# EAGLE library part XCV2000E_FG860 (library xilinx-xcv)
xcv2000e_fg860 edit this description Auto generated by make-symbol-device-package-bsdl.ulp Rev. 26 Source: xcv2000e_fg860.bsd
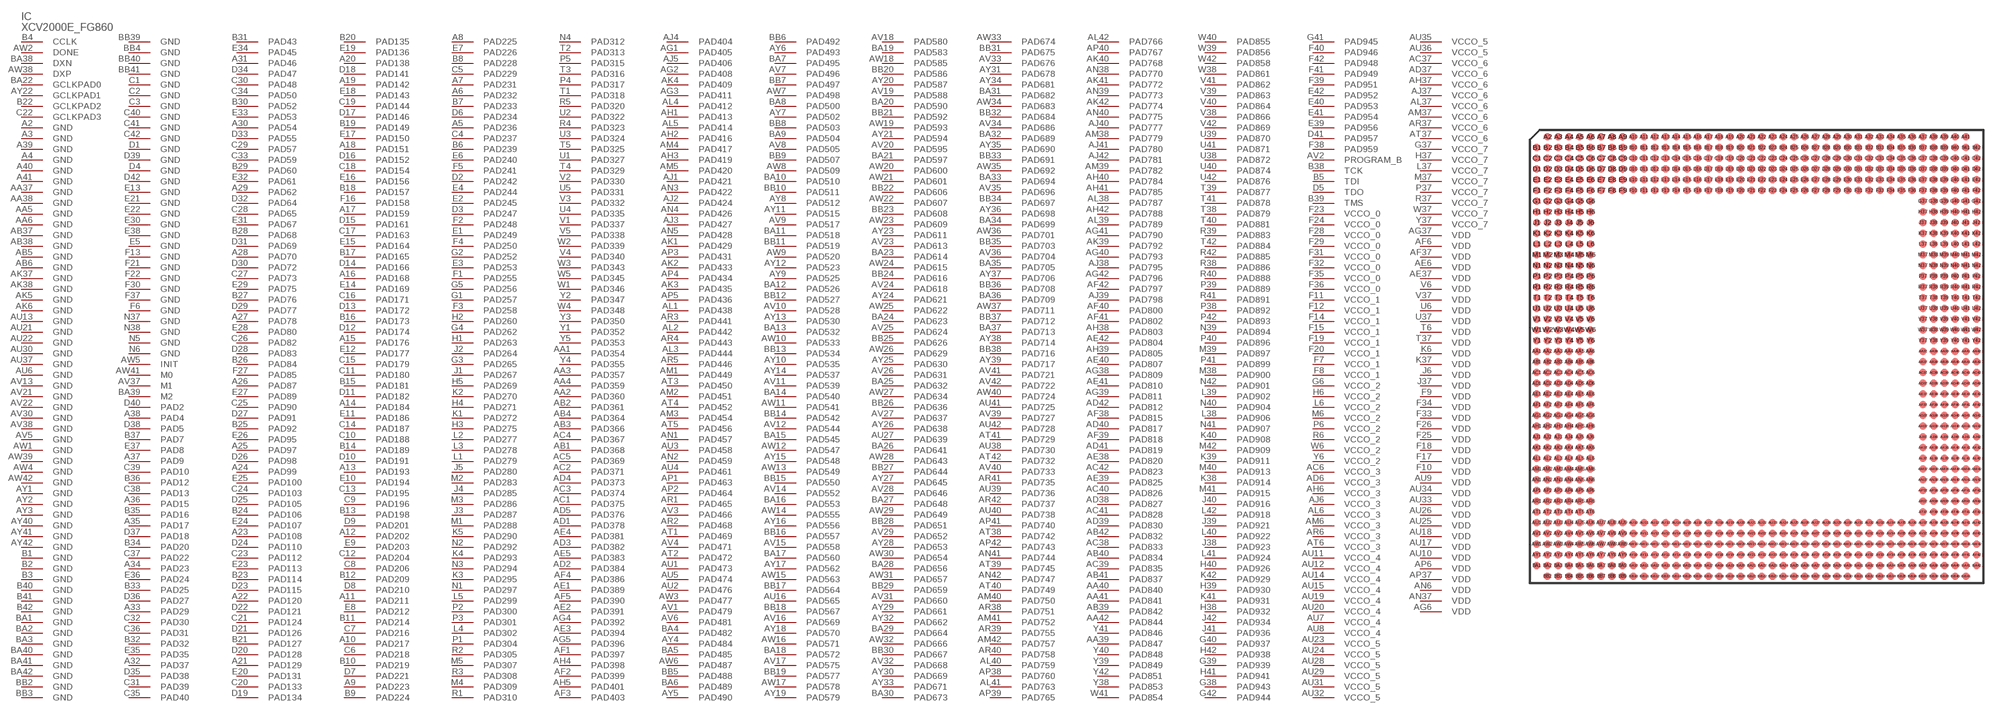
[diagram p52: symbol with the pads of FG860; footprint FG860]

Designator prefix IC

## XCV2000E_FG860 (OC_FARNELL: unknown; OC_NEWARK: unknown)  [FG860]
A2  GND  pwr
A3  GND  pwr
A4  GND  pwr
A5  PAD236
A6  PAD232
A7  PAD231
A8  PAD225
A9  PAD223
A10  PAD217
A11  PAD211
A12  PAD202
A13  PAD193
A14  PAD184
A15  PAD176
A16  PAD168
A17  PAD159
A18  PAD151
A19  PAD142
A20  PAD138
A21  PAD129
A22  PAD120
A23  PAD108
A24  PAD99
A25  PAD97
A26  PAD87
A27  PAD78
A28  PAD70
A29  PAD62
A30  PAD54
A31  PAD46
A32  PAD37
A33  PAD29
A34  PAD23
A35  PAD17
A36  PAD15
A37  PAD9
A38  PAD4
A39  GND  pwr
A40  GND  pwr
A41  GND  pwr
AA1  PAD354
AA2  PAD360
AA3  PAD357
AA4  PAD359
AA5  GND  pwr
AA6  GND  pwr
AA37  GND  pwr
AA38  GND  pwr
AA39  PAD847
AA40  PAD840
AA41  PAD841
AA42  PAD844
AB1  PAD368
AB2  PAD361
AB3  PAD366
AB4  PAD364
AB5  GND  pwr
AB6  GND  pwr
AB37  GND  pwr
AB38  GND  pwr
AB39  PAD842
AB40  PAD834
AB41  PAD837
AB42  PAD832
AC1  PAD375
AC2  PAD371
AC3  PAD374
AC4  PAD367
AC5  PAD369
AC6  VCCO_3  pwr
AC37  VCCO_6  pwr
AC38  PAD833
AC39  PAD835
AC40  PAD826
AC41  PAD828
AC42  PAD823
AD1  PAD378
AD2  PAD384
AD3  PAD382
AD4  PAD373
AD5  PAD376
AD6  VCCO_3  pwr
AD37  VCCO_6  pwr
AD38  PAD827
AD39  PAD830
AD40  PAD817
AD41  PAD819
AD42  PAD812
AE1  PAD389
AE2  PAD391
AE3  PAD394
AE4  PAD381
AE5  PAD383
AE6  VDD  pwr
AE37  VDD  pwr
AE38  PAD820
AE39  PAD825
AE40  PAD807
AE41  PAD810
AE42  PAD804
AF1  PAD397
AF2  PAD399
AF3  PAD403
AF4  PAD386
AF5  PAD390
AF6  VDD  pwr
AF37  VDD  pwr
AF38  PAD815
AF39  PAD818
AF40  PAD800
AF41  PAD802
AF42  PAD797
AG1  PAD405
AG2  PAD408
AG3  PAD411
AG4  PAD392
AG5  PAD396
AG6  VDD  pwr
AG37  VDD  pwr
AG38  PAD809
AG39  PAD811
AG40  PAD793
AG41  PAD790
AG42  PAD796
AH1  PAD413
AH2  PAD416
AH3  PAD419
AH4  PAD398
AH5  PAD401
AH6  VCCO_3  pwr
AH37  VCCO_6  pwr
AH38  PAD803
AH39  PAD805
AH40  PAD784
AH41  PAD785
AH42  PAD788
AJ1  PAD421
AJ2  PAD424
AJ3  PAD427
AJ4  PAD404
AJ5  PAD406
AJ6  VCCO_3  pwr
AJ37  VCCO_6  pwr
AJ38  PAD795
AJ39  PAD798
AJ40  PAD777
AJ41  PAD780
AJ42  PAD781
AK1  PAD429
AK2  PAD433
AK3  PAD435
AK4  PAD409
AK5  GND  pwr
AK6  GND  pwr
AK37  GND  pwr
AK38  GND  pwr
AK39  PAD792
AK40  PAD768
AK41  PAD772
AK42  PAD774
AL1  PAD438
AL2  PAD442
AL3  PAD444
AL4  PAD412
AL5  PAD414
AL6  VCCO_3  pwr
AL37  VCCO_6  pwr
AL38  PAD787
AL39  PAD789
AL40  PAD759
AL41  PAD763
AL42  PAD766
AM1  PAD449
AM2  PAD451
AM3  PAD454
AM4  PAD417
AM5  PAD420
AM6  VCCO_3  pwr
AM37  VCCO_6  pwr
AM38  PAD779
AM39  PAD782
AM40  PAD750
AM41  PAD752
AM42  PAD757
AN1  PAD457
AN2  PAD459
AN3  PAD422
AN4  PAD426
AN5  PAD428
AN6  VDD  pwr
AN37  VDD  pwr
AN38  PAD770
AN39  PAD773
AN40  PAD775
AN41  PAD744
AN42  PAD747
AP1  PAD463
AP2  PAD464
AP3  PAD431
AP4  PAD434
AP5  PAD436
AP6  VDD  pwr
AP37  VDD  pwr
AP38  PAD760
AP39  PAD765
AP40  PAD767
AP41  PAD740
AP42  PAD743
AR1  PAD465
AR2  PAD468
AR3  PAD441
AR4  PAD443
AR5  PAD446
AR6  VCCO_3  pwr
AR37  VCCO_6  pwr
AR38  PAD751
AR39  PAD755
AR40  PAD758
AR41  PAD735
AR42  PAD737
AT1  PAD469
AT2  PAD472
AT3  PAD450
AT4  PAD452
AT5  PAD456
AT6  VCCO_3  pwr
AT37  VCCO_6  pwr
AT38  PAD742
AT39  PAD745
AT40  PAD749
AT41  PAD729
AT42  PAD732
AU1  PAD473
AU2  PAD476
AU3  PAD458
AU4  PAD461
AU5  PAD474
AU6  GND  pwr
AU7  VCCO_4  pwr
AU8  VCCO_4  pwr
AU9  VDD  pwr
AU10  VDD  pwr
AU11  VCCO_4  pwr
AU12  VCCO_4  pwr
AU13  GND  pwr
AU14  VCCO_4  pwr
AU15  VCCO_4  pwr
AU16  PAD565
AU17  VDD  pwr
AU18  VDD  pwr
AU19  VCCO_4  pwr
AU20  VCCO_4  pwr
AU21  GND  pwr
AU22  GND  pwr
AU23  VCCO_5  pwr
AU24  VCCO_5  pwr
AU25  VDD  pwr
AU26  VDD  pwr
AU27  PAD639
AU28  VCCO_5  pwr
AU29  VCCO_5  pwr
AU30  GND  pwr
AU31  VCCO_5  pwr
AU32  VCCO_5  pwr
AU33  VDD  pwr
AU34  VDD  pwr
AU35  VCCO_5  pwr
AU36  VCCO_5  pwr
AU37  GND  pwr
AU38  PAD730
AU39  PAD736
AU40  PAD738
AU41  PAD725
AU42  PAD728
AV1  PAD479
AV2  PROGRAM_B  in
AV3  PAD466
AV4  PAD471
AV5  GND  pwr
AV6  PAD481
AV7  PAD496
AV8  PAD505
AV9  PAD517
AV10  PAD528
AV11  PAD539
AV12  PAD544
AV13  GND  pwr
AV14  PAD552
AV15  PAD558
AV16  PAD569
AV17  PAD575
AV18  PAD580
AV19  PAD588
AV20  PAD595
AV21  GND  pwr
AV22  GND  pwr
AV23  PAD613
AV24  PAD618
AV25  PAD624
AV26  PAD631
AV27  PAD637
AV28  PAD646
AV29  PAD652
AV30  GND  pwr
AV31  PAD660
AV32  PAD668
AV33  PAD676
AV34  PAD686
AV35  PAD696
AV36  PAD704
AV37  M1  in
AV38  GND  pwr
AV39  PAD727
AV40  PAD733
AV41  PAD721
AV42  PAD722
AW1  GND  pwr
AW2  DONE
AW3  PAD477
AW4  GND  pwr
AW5  INIT
AW6  PAD487
AW7  PAD498
AW8  PAD509
AW9  PAD520
AW10  PAD533
AW11  PAD541
AW12  PAD547
AW13  PAD549
AW14  PAD555
AW15  PAD563
AW16  PAD571
AW17  PAD578
AW18  PAD585
AW19  PAD593
AW20  PAD600
AW21  PAD601
AW22  PAD607
AW23  PAD609
AW24  PAD615
AW25  PAD622
AW26  PAD629
AW27  PAD634
AW28  PAD643
AW29  PAD649
AW30  PAD654
AW31  PAD657
AW32  PAD666
AW33  PAD674
AW34  PAD683
AW35  PAD692
AW36  PAD701
AW37  PAD711
AW38  DXP  pas
AW39  GND  pwr
AW40  PAD724
AW41  M0  in
AW42  GND  pwr
AY1  GND  pwr
AY2  GND  pwr
AY3  GND  pwr
AY4  PAD484
AY5  PAD490
AY6  PAD493
AY7  PAD502
AY8  PAD512
AY9  PAD525
AY10  PAD535
AY11  PAD515
AY12  PAD523
AY13  PAD530
AY14  PAD537
AY15  PAD548
AY16  PAD556
AY17  PAD562
AY18  PAD570
AY19  PAD579
AY20  PAD587
AY21  PAD594
AY22  GCLKPAD1  in
AY23  PAD611
AY24  PAD621
AY25  PAD630
AY26  PAD638
AY27  PAD645
AY28  PAD653
AY29  PAD661
AY30  PAD669
AY31  PAD678
AY32  PAD662
AY33  PAD671
AY34  PAD681
AY35  PAD690
AY36  PAD698
AY37  PAD706
AY38  PAD714
AY39  PAD717
AY40  GND  pwr
AY41  GND  pwr
AY42  GND  pwr
B1  GND  pwr
B2  GND  pwr
B3  GND  pwr
B4  CCLK
B5  TDI  in
B6  PAD239
B7  PAD233
B8  PAD228
B9  PAD224
B10  PAD219
B11  PAD214
B12  PAD209
B13  PAD198
B14  PAD189
B15  PAD181
B16  PAD173
B17  PAD165
B18  PAD157
B19  PAD149
B20  PAD135
B21  PAD127
B22  GCLKPAD2  in
B23  PAD114
B24  PAD106
B25  PAD92
B26  PAD84
B27  PAD76
B28  PAD68
B29  PAD60
B30  PAD52
B31  PAD43
B32  PAD32
B33  PAD25
B34  PAD20
B35  PAD16
B36  PAD12
B37  PAD7
B38  TCK  in
B39  TMS  in
B40  GND  pwr
B41  GND  pwr
B42  GND  pwr
BA1  GND  pwr
BA2  GND  pwr
BA3  GND  pwr
BA4  PAD482
BA5  PAD485
BA6  PAD489
BA7  PAD495
BA8  PAD500
BA9  PAD504
BA10  PAD510
BA11  PAD518
BA12  PAD526
BA13  PAD532
BA14  PAD540
BA15  PAD545
BA16  PAD553
BA17  PAD560
BA18  PAD572
BA19  PAD583
BA20  PAD590
BA21  PAD597
BA22  GCLKPAD0  in
BA23  PAD614
BA24  PAD623
BA25  PAD632
BA26  PAD641
BA27  PAD648
BA28  PAD656
BA29  PAD664
BA30  PAD673
BA31  PAD682
BA32  PAD689
BA33  PAD694
BA34  PAD699
BA35  PAD705
BA36  PAD709
BA37  PAD713
BA38  DXN  pas
BA39  M2  in
BA40  GND  pwr
BA41  GND  pwr
BA42  GND  pwr
BB2  GND  pwr
BB3  GND  pwr
BB4  GND  pwr
BB5  PAD488
BB6  PAD492
BB7  PAD497
BB8  PAD503
BB9  PAD507
BB10  PAD511
BB11  PAD519
BB12  PAD527
BB13  PAD534
BB14  PAD542
BB15  PAD550
BB16  PAD557
BB17  PAD564
BB18  PAD567
BB19  PAD577
BB20  PAD586
BB21  PAD592
BB22  PAD606
BB23  PAD608
BB24  PAD616
BB25  PAD626
BB26  PAD636
BB27  PAD644
BB28  PAD651
BB29  PAD659
BB30  PAD667
BB31  PAD675
BB32  PAD684
BB33  PAD691
BB34  PAD697
BB35  PAD703
BB36  PAD708
BB37  PAD712
BB38  PAD716
BB39  GND  pwr
BB40  GND  pwr
BB41  GND  pwr
C1  GND  pwr
C2  GND  pwr
C3  GND  pwr
C4  PAD237
C5  PAD229
C6  PAD218
C7  PAD216
C8  PAD206
C9  PAD196
C10  PAD188
C11  PAD180
C12  PAD204
C13  PAD195
C14  PAD187
C15  PAD179
C16  PAD171
C17  PAD163
C18  PAD154
C19  PAD144
C20  PAD133
C21  PAD124
C22  GCLKPAD3  in
C23  PAD112
C24  PAD103
C25  PAD90
C26  PAD82
C27  PAD73
C28  PAD65
C29  PAD57
C30  PAD48
C31  PAD39
C32  PAD30
C33  PAD59
C34  PAD50
C35  PAD40
C36  PAD31
C37  PAD22
C38  PAD13
C39  PAD10
C40  GND  pwr
C41  GND  pwr
C42  GND  pwr
D1  GND  pwr
D2  PAD242
D3  PAD247
D4  GND  pwr
D5  TDO  out
D6  PAD234
D7  PAD221
D8  PAD210
D9  PAD201
D10  PAD191
D11  PAD182
D12  PAD174
D13  PAD172
D14  PAD166
D15  PAD161
D16  PAD152
D17  PAD146
D18  PAD141
D19  PAD134
D20  PAD128
D21  PAD126
D22  PAD121
D23  PAD115
D24  PAD110
D25  PAD105
D26  PAD98
D27  PAD91
D28  PAD83
D29  PAD77
D30  PAD72
D31  PAD69
D32  PAD64
D33  PAD55
D34  PAD47
D35  PAD38
D36  PAD27
D37  PAD18
D38  PAD5
D39  GND  pwr
D40  PAD2
D41  PAD957
D42  GND  pwr
E1  PAD249
E2  PAD245
E3  PAD253
E4  PAD244
E5  GND  pwr
E6  PAD240
E7  PAD226
E8  PAD212
E9  PAD203
E10  PAD194
E11  PAD186
E12  PAD177
E13  GND  pwr
E14  PAD169
E15  PAD164
E16  PAD156
E17  PAD150
E18  PAD143
E19  PAD136
E20  PAD131
E21  GND  pwr
E22  GND  pwr
E23  PAD113
E24  PAD107
E25  PAD100
E26  PAD95
E27  PAD89
E28  PAD80
E29  PAD75
E30  GND  pwr
E31  PAD67
E32  PAD61
E33  PAD53
E34  PAD45
E35  PAD35
E36  PAD24
E37  PAD8
E38  GND  pwr
E39  PAD956
E40  PAD953
E41  PAD954
E42  PAD952
F1  PAD255
F2  PAD248
F3  PAD258
F4  PAD250
F5  PAD241
F6  GND  pwr
F7  VCCO_1  pwr
F8  VCCO_1  pwr
F9  VDD  pwr
F10  VDD  pwr
F11  VCCO_1  pwr
F12  VCCO_1  pwr
F13  GND  pwr
F14  VCCO_1  pwr
F15  VCCO_1  pwr
F16  PAD158
F17  VDD  pwr
F18  VDD  pwr
F19  VCCO_1  pwr
F20  VCCO_1  pwr
F21  GND  pwr
F22  GND  pwr
F23  VCCO_0  pwr
F24  VCCO_0  pwr
F25  VDD  pwr
F26  VDD  pwr
F27  PAD85
F28  VCCO_0  pwr
F29  VCCO_0  pwr
F30  GND  pwr
F31  VCCO_0  pwr
F32  VCCO_0  pwr
F33  VDD  pwr
F34  VDD  pwr
F35  VCCO_0  pwr
F36  VCCO_0  pwr
F37  GND  pwr
F38  PAD959
F39  PAD951
F40  PAD946
F41  PAD949
F42  PAD948
G1  PAD257
G2  PAD252
G3  PAD265
G4  PAD262
G5  PAD256
G6  VCCO_2  pwr
G37  VCCO_7  pwr
G38  PAD943
G39  PAD939
G40  PAD937
G41  PAD945
G42  PAD944
H1  PAD263
H2  PAD260
H3  PAD275
H4  PAD271
H5  PAD269
H6  VCCO_2  pwr
H37  VCCO_7  pwr
H38  PAD932
H39  PAD930
H40  PAD926
H41  PAD941
H42  PAD938
J1  PAD267
J2  PAD264
J3  PAD287
J4  PAD285
J5  PAD280
J6  VDD  pwr
J37  VDD  pwr
J38  PAD923
J39  PAD921
J40  PAD916
J41  PAD936
J42  PAD934
K1  PAD272
K2  PAD270
K3  PAD295
K4  PAD293
K5  PAD290
K6  VDD  pwr
K37  VDD  pwr
K38  PAD914
K39  PAD911
K40  PAD908
K41  PAD931
K42  PAD929
L1  PAD279
L2  PAD277
L3  PAD278
L4  PAD302
L5  PAD299
L6  VCCO_2  pwr
L37  VCCO_7  pwr
L38  PAD906
L39  PAD902
L40  PAD922
L41  PAD924
L42  PAD918
M1  PAD288
M2  PAD283
M3  PAD286
M4  PAD309
M5  PAD307
M6  VCCO_2  pwr
M37  VCCO_7  pwr
M38  PAD900
M39  PAD897
M40  PAD913
M41  PAD915
M42  PAD909
N1  PAD297
N2  PAD292
N3  PAD294
N4  PAD312
N5  GND  pwr
N6  GND  pwr
N37  GND  pwr
N38  GND  pwr
N39  PAD894
N40  PAD904
N41  PAD907
N42  PAD901
P1  PAD304
P2  PAD300
P3  PAD301
P4  PAD317
P5  PAD315
P6  VCCO_2  pwr
P37  VCCO_7  pwr
P38  PAD892
P39  PAD889
P40  PAD896
P41  PAD899
P42  PAD893
R1  PAD310
R2  PAD305
R3  PAD308
R4  PAD323
R5  PAD320
R6  VCCO_2  pwr
R37  VCCO_7  pwr
R38  PAD886
R39  PAD883
R40  PAD888
R41  PAD891
R42  PAD885
T1  PAD318
T2  PAD313
T3  PAD316
T4  PAD329
T5  PAD325
T6  VDD  pwr
T37  VDD  pwr
T38  PAD879
T39  PAD877
T40  PAD881
T41  PAD878
T42  PAD884
U1  PAD327
U2  PAD322
U3  PAD324
U4  PAD335
U5  PAD331
U6  VDD  pwr
U37  VDD  pwr
U38  PAD872
U39  PAD870
U40  PAD874
U41  PAD871
U42  PAD876
V1  PAD337
V2  PAD330
V3  PAD332
V4  PAD340
V5  PAD338
V6  VDD  pwr
V37  VDD  pwr
V38  PAD866
V39  PAD863
V40  PAD864
V41  PAD862
V42  PAD869
W1  PAD346
W2  PAD339
W3  PAD343
W4  PAD348
W5  PAD345
W6  VCCO_2  pwr
W37  VCCO_7  pwr
W38  PAD861
W39  PAD856
W40  PAD855
W41  PAD854
W42  PAD858
Y1  PAD352
Y2  PAD347
Y3  PAD350
Y4  PAD355
Y5  PAD353
Y6  VCCO_2  pwr
Y37  VCCO_7  pwr
Y38  PAD853
Y39  PAD849
Y40  PAD848
Y41  PAD846
Y42  PAD851

## Footprint FG860 (pad centres in mm)
xcv1000e_fg860_1532 edit this description Auto generated by make-symbol-device-package-bsdl.ulp Rev. 26 Source: xcv1000e_fg860_1532.bsd
smd 0.7 x 0.7: A2 -19.5,20.5; A3 -18.5,20.5; A4 -17.5,20.5; A5 -16.5,20.5; A6 -15.5,20.5; A7 -14.5,20.5; A8 -13.5,20.5; A9 -12.5,20.5; A10 -11.5,20.5; A11 -10.5,20.5; A12 -9.5,20.5; A13 -8.5,20.5; A14 -7.5,20.5; A15 -6.5,20.5; A16 -5.5,20.5; A17 -4.5,20.5; A18 -3.5,20.5; A19 -2.5,20.5; A20 -1.5,20.5; A21 -0.5,20.5; A22 0.5,20.5; A23 1.5,20.5; A24 2.5,20.5; A25 3.5,20.5; A26 4.5,20.5; A27 5.5,20.5; A28 6.5,20.5; A29 7.5,20.5; A30 8.5,20.5; A31 9.5,20.5; A32 10.5,20.5; A33 11.5,20.5; A34 12.5,20.5; A35 13.5,20.5; A36 14.5,20.5; A37 15.5,20.5; A38 16.5,20.5; A39 17.5,20.5; A40 18.5,20.5; A41 19.5,20.5; AA1 -20.5,0.5; AA2 -19.5,0.5; AA3 -18.5,0.5; AA4 -17.5,0.5; AA5 -16.5,0.5; AA6 -15.5,0.5; AA37 15.5,0.5; AA38 16.5,0.5; AA39 17.5,0.5; AA40 18.5,0.5; AA41 19.5,0.5; AA42 20.5,0.5; AB1 -20.5,-0.5; AB2 -19.5,-0.5; AB3 -18.5,-0.5; AB4 -17.5,-0.5; AB5 -16.5,-0.5; AB6 -15.5,-0.5; AB37 15.5,-0.5; AB38 16.5,-0.5; AB39 17.5,-0.5; AB40 18.5,-0.5; AB41 19.5,-0.5; AB42 20.5,-0.5; AC1 -20.5,-1.5; AC2 -19.5,-1.5; AC3 -18.5,-1.5; AC4 -17.5,-1.5; AC5 -16.5,-1.5; AC6 -15.5,-1.5; AC37 15.5,-1.5; AC38 16.5,-1.5; AC39 17.5,-1.5; AC40 18.5,-1.5; AC41 19.5,-1.5; AC42 20.5,-1.5; AD1 -20.5,-2.5; AD2 -19.5,-2.5; AD3 -18.5,-2.5; AD4 -17.5,-2.5; AD5 -16.5,-2.5; AD6 -15.5,-2.5; AD37 15.5,-2.5; AD38 16.5,-2.5; AD39 17.5,-2.5; AD40 18.5,-2.5; AD41 19.5,-2.5; AD42 20.5,-2.5; AE1 -20.5,-3.5; AE2 -19.5,-3.5; AE3 -18.5,-3.5; AE4 -17.5,-3.5; AE5 -16.5,-3.5; AE6 -15.5,-3.5; AE37 15.5,-3.5; AE38 16.5,-3.5; AE39 17.5,-3.5; AE40 18.5,-3.5; AE41 19.5,-3.5; AE42 20.5,-3.5; AF1 -20.5,-4.5; AF2 -19.5,-4.5; AF3 -18.5,-4.5; AF4 -17.5,-4.5; AF5 -16.5,-4.5; AF6 -15.5,-4.5; AF37 15.5,-4.5; AF38 16.5,-4.5; AF39 17.5,-4.5; AF40 18.5,-4.5; AF41 19.5,-4.5; AF42 20.5,-4.5; AG1 -20.5,-5.5; AG2 -19.5,-5.5; AG3 -18.5,-5.5; AG4 -17.5,-5.5; AG5 -16.5,-5.5; AG6 -15.5,-5.5; AG37 15.5,-5.5; AG38 16.5,-5.5; AG39 17.5,-5.5; AG40 18.5,-5.5; AG41 19.5,-5.5; AG42 20.5,-5.5; AH1 -20.5,-6.5; AH2 -19.5,-6.5; AH3 -18.5,-6.5; AH4 -17.5,-6.5; AH5 -16.5,-6.5; AH6 -15.5,-6.5; AH37 15.5,-6.5; AH38 16.5,-6.5; AH39 17.5,-6.5; AH40 18.5,-6.5; AH41 19.5,-6.5; AH42 20.5,-6.5; AJ1 -20.5,-7.5; AJ2 -19.5,-7.5; AJ3 -18.5,-7.5; AJ4 -17.5,-7.5; AJ5 -16.5,-7.5; AJ6 -15.5,-7.5; AJ37 15.5,-7.5; AJ38 16.5,-7.5; AJ39 17.5,-7.5; AJ40 18.5,-7.5; AJ41 19.5,-7.5; AJ42 20.5,-7.5; AK1 -20.5,-8.5; AK2 -19.5,-8.5; AK3 -18.5,-8.5; AK4 -17.5,-8.5; AK5 -16.5,-8.5; AK6 -15.5,-8.5; AK37 15.5,-8.5; AK38 16.5,-8.5; AK39 17.5,-8.5; AK40 18.5,-8.5; AK41 19.5,-8.5; AK42 20.5,-8.5; AL1 -20.5,-9.5; AL2 -19.5,-9.5; AL3 -18.5,-9.5; AL4 -17.5,-9.5; AL5 -16.5,-9.5; AL6 -15.5,-9.5; AL37 15.5,-9.5; AL38 16.5,-9.5; AL39 17.5,-9.5; AL40 18.5,-9.5; AL41 19.5,-9.5; AL42 20.5,-9.5; AM1 -20.5,-10.5; AM2 -19.5,-10.5; AM3 -18.5,-10.5; AM4 -17.5,-10.5; AM5 -16.5,-10.5; AM6 -15.5,-10.5; AM37 15.5,-10.5; AM38 16.5,-10.5; AM39 17.5,-10.5; AM40 18.5,-10.5; AM41 19.5,-10.5; AM42 20.5,-10.5; AN1 -20.5,-11.5; AN2 -19.5,-11.5; AN3 -18.5,-11.5; AN4 -17.5,-11.5; AN5 -16.5,-11.5; AN6 -15.5,-11.5; AN37 15.5,-11.5; AN38 16.5,-11.5; AN39 17.5,-11.5; AN40 18.5,-11.5; AN41 19.5,-11.5; AN42 20.5,-11.5; AP1 -20.5,-12.5; AP2 -19.5,-12.5; AP3 -18.5,-12.5; AP4 -17.5,-12.5; AP5 -16.5,-12.5; AP6 -15.5,-12.5; AP37 15.5,-12.5; AP38 16.5,-12.5; AP39 17.5,-12.5; AP40 18.5,-12.5; AP41 19.5,-12.5; AP42 20.5,-12.5; AR1 -20.5,-13.5; AR2 -19.5,-13.5; AR3 -18.5,-13.5; AR4 -17.5,-13.5; AR5 -16.5,-13.5; AR6 -15.5,-13.5; AR37 15.5,-13.5; AR38 16.5,-13.5; AR39 17.5,-13.5; AR40 18.5,-13.5; AR41 19.5,-13.5; AR42 20.5,-13.5; AT1 -20.5,-14.5; AT2 -19.5,-14.5; AT3 -18.5,-14.5; AT4 -17.5,-14.5; AT5 -16.5,-14.5; AT6 -15.5,-14.5; AT37 15.5,-14.5; AT38 16.5,-14.5; AT39 17.5,-14.5; AT40 18.5,-14.5; AT41 19.5,-14.5; AT42 20.5,-14.5; AU1 -20.5,-15.5; AU2 -19.5,-15.5; AU3 -18.5,-15.5; AU4 -17.5,-15.5; AU5 -16.5,-15.5; AU6 -15.5,-15.5; AU7 -14.5,-15.5; AU8 -13.5,-15.5; AU9 -12.5,-15.5; AU10 -11.5,-15.5; AU11 -10.5,-15.5; AU12 -9.5,-15.5; AU13 -8.5,-15.5; AU14 -7.5,-15.5; AU15 -6.5,-15.5; AU16 -5.5,-15.5; AU17 -4.5,-15.5; AU18 -3.5,-15.5; AU19 -2.5,-15.5; AU20 -1.5,-15.5; AU21 -0.5,-15.5; AU22 0.5,-15.5; AU23 1.5,-15.5; AU24 2.5,-15.5; AU25 3.5,-15.5; AU26 4.5,-15.5; AU27 5.5,-15.5; AU28 6.5,-15.5; AU29 7.5,-15.5; AU30 8.5,-15.5; AU31 9.5,-15.5; AU32 10.5,-15.5; AU33 11.5,-15.5; AU34 12.5,-15.5; AU35 13.5,-15.5; AU36 14.5,-15.5; AU37 15.5,-15.5; AU38 16.5,-15.5; AU39 17.5,-15.5; AU40 18.5,-15.5; AU41 19.5,-15.5; AU42 20.5,-15.5; AV1 -20.5,-16.5; AV2 -19.5,-16.5; AV3 -18.5,-16.5; AV4 -17.5,-16.5; AV5 -16.5,-16.5; AV6 -15.5,-16.5; AV7 -14.5,-16.5; AV8 -13.5,-16.5; AV9 -12.5,-16.5; AV10 -11.5,-16.5; AV11 -10.5,-16.5; AV12 -9.5,-16.5; AV13 -8.5,-16.5; AV14 -7.5,-16.5; AV15 -6.5,-16.5; AV16 -5.5,-16.5; AV17 -4.5,-16.5; AV18 -3.5,-16.5; AV19 -2.5,-16.5; AV20 -1.5,-16.5; AV21 -0.5,-16.5; AV22 0.5,-16.5; AV23 1.5,-16.5; AV24 2.5,-16.5; AV25 3.5,-16.5; AV26 4.5,-16.5; AV27 5.5,-16.5; AV28 6.5,-16.5; AV29 7.5,-16.5; AV30 8.5,-16.5; AV31 9.5,-16.5; AV32 10.5,-16.5; AV33 11.5,-16.5; AV34 12.5,-16.5; AV35 13.5,-16.5; AV36 14.5,-16.5; AV37 15.5,-16.5; AV38 16.5,-16.5; AV39 17.5,-16.5; AV40 18.5,-16.5; AV41 19.5,-16.5; AV42 20.5,-16.5; AW1 -20.5,-17.5; AW2 -19.5,-17.5; AW3 -18.5,-17.5; AW4 -17.5,-17.5; AW5 -16.5,-17.5; AW6 -15.5,-17.5; AW7 -14.5,-17.5; AW8 -13.5,-17.5; AW9 -12.5,-17.5; AW10 -11.5,-17.5; AW11 -10.5,-17.5; AW12 -9.5,-17.5; AW13 -8.5,-17.5; AW14 -7.5,-17.5; AW15 -6.5,-17.5; AW16 -5.5,-17.5; AW17 -4.5,-17.5; AW18 -3.5,-17.5; AW19 -2.5,-17.5; AW20 -1.5,-17.5; AW21 -0.5,-17.5; AW22 0.5,-17.5; AW23 1.5,-17.5; AW24 2.5,-17.5; AW25 3.5,-17.5; AW26 4.5,-17.5; AW27 5.5,-17.5; AW28 6.5,-17.5; AW29 7.5,-17.5; AW30 8.5,-17.5; AW31 9.5,-17.5; AW32 10.5,-17.5; AW33 11.5,-17.5; AW34 12.5,-17.5; AW35 13.5,-17.5; AW36 14.5,-17.5; AW37 15.5,-17.5; AW38 16.5,-17.5; AW39 17.5,-17.5; AW40 18.5,-17.5; AW41 19.5,-17.5; AW42 20.5,-17.5; AY1 -20.5,-18.5; AY2 -19.5,-18.5; AY3 -18.5,-18.5; AY4 -17.5,-18.5; AY5 -16.5,-18.5; AY6 -15.5,-18.5; AY7 -14.5,-18.5; AY8 -13.5,-18.5; AY9 -12.5,-18.5; AY10 -11.5,-18.5; AY11 -10.5,-18.5; AY12 -9.5,-18.5; AY13 -8.5,-18.5; AY14 -7.5,-18.5; AY15 -6.5,-18.5; AY16 -5.5,-18.5; AY17 -4.5,-18.5; AY18 -3.5,-18.5; AY19 -2.5,-18.5; AY20 -1.5,-18.5; AY21 -0.5,-18.5; AY22 0.5,-18.5; AY23 1.5,-18.5; AY24 2.5,-18.5; AY25 3.5,-18.5; AY26 4.5,-18.5; AY27 5.5,-18.5; AY28 6.5,-18.5; AY29 7.5,-18.5; AY30 8.5,-18.5; AY31 9.5,-18.5; AY32 10.5,-18.5; AY33 11.5,-18.5; AY34 12.5,-18.5; AY35 13.5,-18.5; AY36 14.5,-18.5; AY37 15.5,-18.5; AY38 16.5,-18.5; AY39 17.5,-18.5; AY40 18.5,-18.5; AY41 19.5,-18.5; AY42 20.5,-18.5; B1 -20.5,19.5; B2 -19.5,19.5; B3 -18.5,19.5; B4 -17.5,19.5; B5 -16.5,19.5; B6 -15.5,19.5; B7 -14.5,19.5; B8 -13.5,19.5; B9 -12.5,19.5; B10 -11.5,19.5; B11 -10.5,19.5; B12 -9.5,19.5; B13 -8.5,19.5; B14 -7.5,19.5; B15 -6.5,19.5; B16 -5.5,19.5; B17 -4.5,19.5; B18 -3.5,19.5; B19 -2.5,19.5; B20 -1.5,19.5; B21 -0.5,19.5; B22 0.5,19.5; B23 1.5,19.5; B24 2.5,19.5; B25 3.5,19.5; B26 4.5,19.5; B27 5.5,19.5; B28 6.5,19.5; B29 7.5,19.5; B30 8.5,19.5; B31 9.5,19.5; B32 10.5,19.5; B33 11.5,19.5; B34 12.5,19.5; B35 13.5,19.5; B36 14.5,19.5; B37 15.5,19.5; B38 16.5,19.5; B39 17.5,19.5; B40 18.5,19.5; B41 19.5,19.5; B42 20.5,19.5; BA1 -20.5,-19.5; BA2 -19.5,-19.5; BA3 -18.5,-19.5; BA4 -17.5,-19.5; BA5 -16.5,-19.5; BA6 -15.5,-19.5; BA7 -14.5,-19.5; BA8 -13.5,-19.5; BA9 -12.5,-19.5; BA10 -11.5,-19.5; BA11 -10.5,-19.5; BA12 -9.5,-19.5; BA13 -8.5,-19.5; BA14 -7.5,-19.5; BA15 -6.5,-19.5; BA16 -5.5,-19.5; BA17 -4.5,-19.5; BA18 -3.5,-19.5; BA19 -2.5,-19.5; BA20 -1.5,-19.5; BA21 -0.5,-19.5; BA22 0.5,-19.5; BA23 1.5,-19.5; BA24 2.5,-19.5; BA25 3.5,-19.5; BA26 4.5,-19.5; BA27 5.5,-19.5; BA28 6.5,-19.5; BA29 7.5,-19.5; BA30 8.5,-19.5; BA31 9.5,-19.5; BA32 10.5,-19.5; BA33 11.5,-19.5; BA34 12.5,-19.5; BA35 13.5,-19.5; BA36 14.5,-19.5; BA37 15.5,-19.5; BA38 16.5,-19.5; BA39 17.5,-19.5; BA40 18.5,-19.5; BA41 19.5,-19.5; BA42 20.5,-19.5; BB2 -19.5,-20.5; BB3 -18.5,-20.5; BB4 -17.5,-20.5; BB5 -16.5,-20.5; BB6 -15.5,-20.5; BB7 -14.5,-20.5; BB8 -13.5,-20.5; BB9 -12.5,-20.5; BB10 -11.5,-20.5; BB11 -10.5,-20.5; BB12 -9.5,-20.5; BB13 -8.5,-20.5; BB14 -7.5,-20.5; BB15 -6.5,-20.5; BB16 -5.5,-20.5; BB17 -4.5,-20.5; BB18 -3.5,-20.5; BB19 -2.5,-20.5; BB20 -1.5,-20.5; BB21 -0.5,-20.5; BB22 0.5,-20.5; BB23 1.5,-20.5; BB24 2.5,-20.5; BB25 3.5,-20.5; BB26 4.5,-20.5; BB27 5.5,-20.5; BB28 6.5,-20.5; BB29 7.5,-20.5; BB30 8.5,-20.5; BB31 9.5,-20.5; BB32 10.5,-20.5; BB33 11.5,-20.5; BB34 12.5,-20.5; BB35 13.5,-20.5; BB36 14.5,-20.5; BB37 15.5,-20.5; BB38 16.5,-20.5; BB39 17.5,-20.5; BB40 18.5,-20.5; BB41 19.5,-20.5; C1 -20.5,18.5; C2 -19.5,18.5; C3 -18.5,18.5; C4 -17.5,18.5; C5 -16.5,18.5; C6 -15.5,18.5; C7 -14.5,18.5; C8 -13.5,18.5; C9 -12.5,18.5; C10 -11.5,18.5; C11 -10.5,18.5; C12 -9.5,18.5; C13 -8.5,18.5; C14 -7.5,18.5; C15 -6.5,18.5; C16 -5.5,18.5; C17 -4.5,18.5; C18 -3.5,18.5; C19 -2.5,18.5; C20 -1.5,18.5; C21 -0.5,18.5; C22 0.5,18.5; C23 1.5,18.5; C24 2.5,18.5; C25 3.5,18.5; C26 4.5,18.5; C27 5.5,18.5; C28 6.5,18.5; C29 7.5,18.5; C30 8.5,18.5; C31 9.5,18.5; C32 10.5,18.5; C33 11.5,18.5; C34 12.5,18.5; C35 13.5,18.5; C36 14.5,18.5; C37 15.5,18.5; C38 16.5,18.5; C39 17.5,18.5; C40 18.5,18.5; C41 19.5,18.5; C42 20.5,18.5; D1 -20.5,17.5; D2 -19.5,17.5; D3 -18.5,17.5; D4 -17.5,17.5; D5 -16.5,17.5; D6 -15.5,17.5; D7 -14.5,17.5; D8 -13.5,17.5; D9 -12.5,17.5; D10 -11.5,17.5; D11 -10.5,17.5; D12 -9.5,17.5; D13 -8.5,17.5; D14 -7.5,17.5; D15 -6.5,17.5; D16 -5.5,17.5; D17 -4.5,17.5; D18 -3.5,17.5; D19 -2.5,17.5; D20 -1.5,17.5; D21 -0.5,17.5; D22 0.5,17.5; D23 1.5,17.5; D24 2.5,17.5; D25 3.5,17.5; D26 4.5,17.5; D27 5.5,17.5; D28 6.5,17.5; D29 7.5,17.5; D30 8.5,17.5; D31 9.5,17.5; D32 10.5,17.5; D33 11.5,17.5; D34 12.5,17.5; D35 13.5,17.5; D36 14.5,17.5; D37 15.5,17.5; D38 16.5,17.5; D39 17.5,17.5; D40 18.5,17.5; D41 19.5,17.5; D42 20.5,17.5; E1 -20.5,16.5; E2 -19.5,16.5; E3 -18.5,16.5; E4 -17.5,16.5; E5 -16.5,16.5; E6 -15.5,16.5; E7 -14.5,16.5; E8 -13.5,16.5; E9 -12.5,16.5; E10 -11.5,16.5; E11 -10.5,16.5; E12 -9.5,16.5; E13 -8.5,16.5; E14 -7.5,16.5; E15 -6.5,16.5; E16 -5.5,16.5; E17 -4.5,16.5; E18 -3.5,16.5; E19 -2.5,16.5; E20 -1.5,16.5; E21 -0.5,16.5; E22 0.5,16.5; E23 1.5,16.5; E24 2.5,16.5; E25 3.5,16.5; E26 4.5,16.5; E27 5.5,16.5; E28 6.5,16.5; E29 7.5,16.5; E30 8.5,16.5; E31 9.5,16.5; E32 10.5,16.5; E33 11.5,16.5; E34 12.5,16.5; E35 13.5,16.5; E36 14.5,16.5; E37 15.5,16.5; E38 16.5,16.5; E39 17.5,16.5; E40 18.5,16.5; E41 19.5,16.5; E42 20.5,16.5; F1 -20.5,15.5; F2 -19.5,15.5; F3 -18.5,15.5; F4 -17.5,15.5; F5 -16.5,15.5; F6 -15.5,15.5; F7 -14.5,15.5; F8 -13.5,15.5; F9 -12.5,15.5; F10 -11.5,15.5; F11 -10.5,15.5; F12 -9.5,15.5; F13 -8.5,15.5; F14 -7.5,15.5; F15 -6.5,15.5; F16 -5.5,15.5; F17 -4.5,15.5; F18 -3.5,15.5; F19 -2.5,15.5; F20 -1.5,15.5; F21 -0.5,15.5; F22 0.5,15.5; F23 1.5,15.5; F24 2.5,15.5; F25 3.5,15.5; F26 4.5,15.5; F27 5.5,15.5; F28 6.5,15.5; F29 7.5,15.5; F30 8.5,15.5; F31 9.5,15.5; F32 10.5,15.5; F33 11.5,15.5; F34 12.5,15.5; F35 13.5,15.5; F36 14.5,15.5; F37 15.5,15.5; F38 16.5,15.5; F39 17.5,15.5; F40 18.5,15.5; F41 19.5,15.5; F42 20.5,15.5; G1 -20.5,14.5; G2 -19.5,14.5; G3 -18.5,14.5; G4 -17.5,14.5; G5 -16.5,14.5; G6 -15.5,14.5; G37 15.5,14.5; G38 16.5,14.5; G39 17.5,14.5; G40 18.5,14.5; G41 19.5,14.5; G42 20.5,14.5; H1 -20.5,13.5; H2 -19.5,13.5; H3 -18.5,13.5; H4 -17.5,13.5; H5 -16.5,13.5; H6 -15.5,13.5; H37 15.5,13.5; H38 16.5,13.5; H39 17.5,13.5; H40 18.5,13.5; H41 19.5,13.5; H42 20.5,13.5; J1 -20.5,12.5; J2 -19.5,12.5; J3 -18.5,12.5; J4 -17.5,12.5; J5 -16.5,12.5; J6 -15.5,12.5; J37 15.5,12.5; J38 16.5,12.5; J39 17.5,12.5; J40 18.5,12.5; J41 19.5,12.5; J42 20.5,12.5; K1 -20.5,11.5; K2 -19.5,11.5; K3 -18.5,11.5; K4 -17.5,11.5; K5 -16.5,11.5; K6 -15.5,11.5; K37 15.5,11.5; K38 16.5,11.5; K39 17.5,11.5; K40 18.5,11.5; K41 19.5,11.5; K42 20.5,11.5; L1 -20.5,10.5; L2 -19.5,10.5; L3 -18.5,10.5; L4 -17.5,10.5; L5 -16.5,10.5; L6 -15.5,10.5; L37 15.5,10.5; L38 16.5,10.5; L39 17.5,10.5; L40 18.5,10.5; L41 19.5,10.5; L42 20.5,10.5; M1 -20.5,9.5; M2 -19.5,9.5; M3 -18.5,9.5; M4 -17.5,9.5; M5 -16.5,9.5; M6 -15.5,9.5; M37 15.5,9.5; M38 16.5,9.5; M39 17.5,9.5; M40 18.5,9.5; M41 19.5,9.5; M42 20.5,9.5; N1 -20.5,8.5; N2 -19.5,8.5; N3 -18.5,8.5; N4 -17.5,8.5; N5 -16.5,8.5; N6 -15.5,8.5; N37 15.5,8.5; N38 16.5,8.5; N39 17.5,8.5; N40 18.5,8.5; N41 19.5,8.5; N42 20.5,8.5; P1 -20.5,7.5; P2 -19.5,7.5; P3 -18.5,7.5; P4 -17.5,7.5; P5 -16.5,7.5; P6 -15.5,7.5; P37 15.5,7.5; P38 16.5,7.5; P39 17.5,7.5; P40 18.5,7.5; P41 19.5,7.5; P42 20.5,7.5; R1 -20.5,6.5; R2 -19.5,6.5; R3 -18.5,6.5; R4 -17.5,6.5; R5 -16.5,6.5; R6 -15.5,6.5; R37 15.5,6.5; R38 16.5,6.5; R39 17.5,6.5; R40 18.5,6.5; R41 19.5,6.5; R42 20.5,6.5; T1 -20.5,5.5; T2 -19.5,5.5; T3 -18.5,5.5; T4 -17.5,5.5; T5 -16.5,5.5; T6 -15.5,5.5; T37 15.5,5.5; T38 16.5,5.5; T39 17.5,5.5; T40 18.5,5.5; T41 19.5,5.5; T42 20.5,5.5; U1 -20.5,4.5; U2 -19.5,4.5; U3 -18.5,4.5; U4 -17.5,4.5; U5 -16.5,4.5; U6 -15.5,4.5; U37 15.5,4.5; U38 16.5,4.5; U39 17.5,4.5; U40 18.5,4.5; U41 19.5,4.5; U42 20.5,4.5; V1 -20.5,3.5; V2 -19.5,3.5; V3 -18.5,3.5; V4 -17.5,3.5; V5 -16.5,3.5; V6 -15.5,3.5; V37 15.5,3.5; V38 16.5,3.5; V39 17.5,3.5; V40 18.5,3.5; V41 19.5,3.5; V42 20.5,3.5; W1 -20.5,2.5; W2 -19.5,2.5; W3 -18.5,2.5; W4 -17.5,2.5; W5 -16.5,2.5; W6 -15.5,2.5; W37 15.5,2.5; W38 16.5,2.5; W39 17.5,2.5; W40 18.5,2.5; W41 19.5,2.5; W42 20.5,2.5; Y1 -20.5,1.5; Y2 -19.5,1.5; Y3 -18.5,1.5; Y4 -17.5,1.5; Y5 -16.5,1.5; Y6 -15.5,1.5; Y37 15.5,1.5; Y38 16.5,1.5; Y39 17.5,1.5; Y40 18.5,1.5; Y41 19.5,1.5; Y42 20.5,1.5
